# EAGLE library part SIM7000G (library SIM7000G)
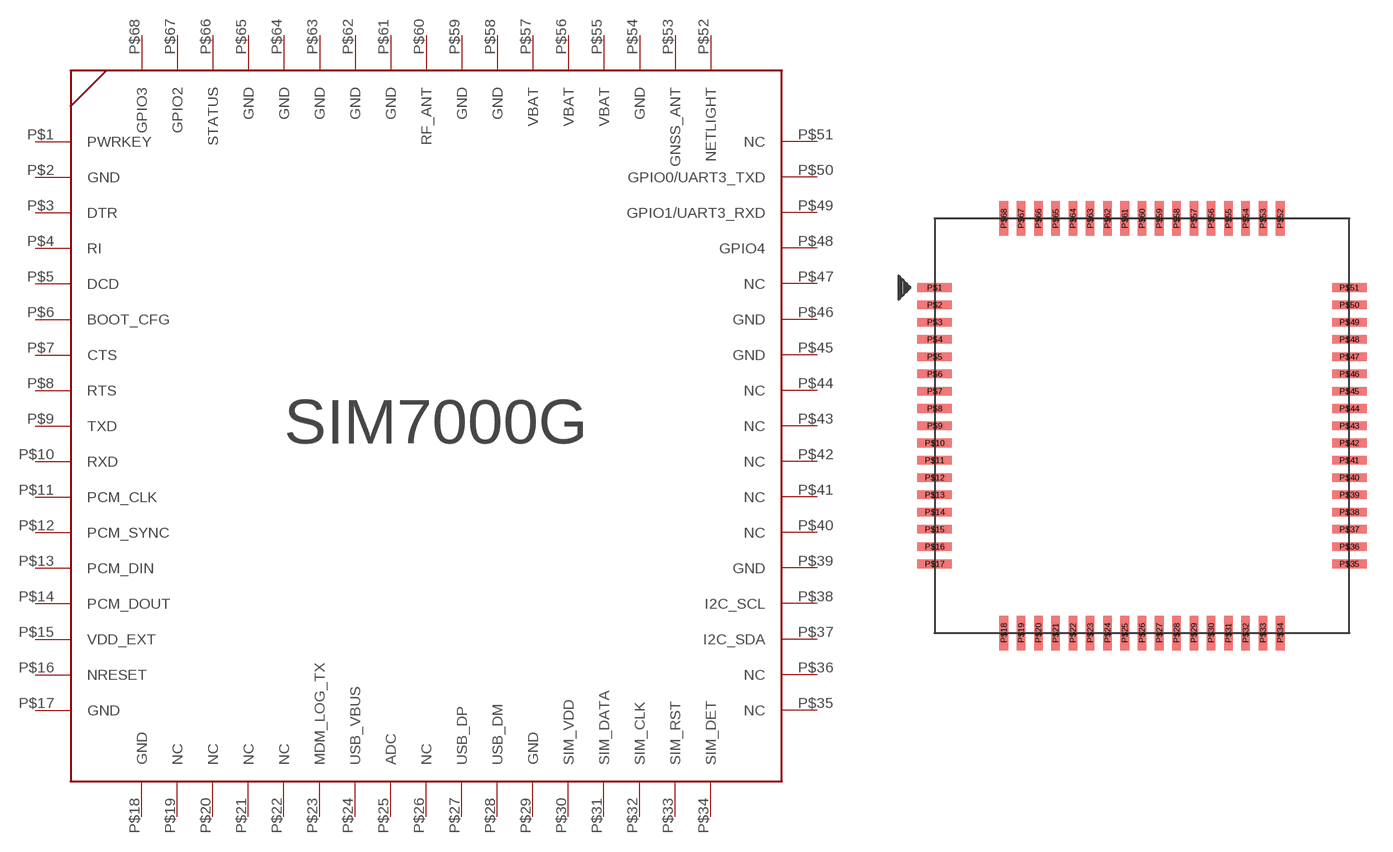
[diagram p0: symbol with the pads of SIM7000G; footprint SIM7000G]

Designator prefix -

## SIM7000G (CHECK_PRICES: https://www.snapeda.com/parts/SIM7000G/SIMCom/view-part/?ref=eda; DESCRIPTION: 802.15.4 Cat-M, Cat-NB, EDGE, GPRS, LPWA Transceiver Module 850MHz, 900MHz, 1.8GHz, 1.9GHz Antenna Not Included Surface Mount; MF: SIMCom Wireless Solutions Limited; MP: SIM7000G; PACKAGE: None; PURCHASE-URL: https://www.snapeda.com/api/url_track_click_mouser/?unipart_id=12130268&manufacturer=SIMCom Wireless Solutions Limited&part_name=SIM7000G&search_term=sim7000g; SNAPEDA_LINK: https://www.snapeda.com/parts/SIM7000G/SIMCom/view-part/?ref=snap)  [SIM7000G]
P$1  PWRKEY
P$2  GND
P$3  DTR
P$4  RI
P$5  DCD
P$6  BOOT_CFG
P$7  CTS
P$8  RTS
P$9  TXD
P$10  RXD
P$11  PCM_CLK
P$12  PCM_SYNC
P$13  PCM_DIN
P$14  PCM_DOUT
P$15  VDD_EXT
P$16  NRESET
P$17  GND
P$18  GND
P$19  NC
P$20  NC
P$21  NC
P$22  NC
P$23  MDM_LOG_TX
P$24  USB_VBUS
P$25  ADC
P$26  NC
P$27  USB_DP
P$28  USB_DM
P$29  GND
P$30  SIM_VDD
P$31  SIM_DATA
P$32  SIM_CLK
P$33  SIM_RST
P$34  SIM_DET
P$35  NC
P$36  NC
P$37  I2C_SDA
P$38  I2C_SCL
P$39  GND
P$40  NC
P$41  NC
P$42  NC
P$43  NC
P$44  NC
P$45  GND
P$46  GND
P$47  NC
P$48  GPIO4
P$49  GPIO1/UART3_RXD
P$50  GPIO0/UART3_TXD
P$51  NC
P$52  NETLIGHT
P$53  GNSS_ANT
P$54  GND
P$55  VBAT
P$56  VBAT
P$57  VBAT
P$58  GND
P$59  GND
P$60  RF_ANT
P$61  GND
P$62  GND
P$63  GND
P$64  GND
P$65  GND
P$66  STATUS
P$67  GPIO2
P$68  GPIO3

## Footprint SIM7000G (pad centres in mm)
smd 2 x 0.5: P$1 -12,8; P$2 -12,7; P$3 -12,6; P$4 -12,5; P$5 -12,4; P$6 -12,3; P$7 -12,2; P$8 -12,1; P$9 -12,0; P$10 -12,-1; P$11 -12,-2; P$12 -12,-3; P$13 -12,-4; P$14 -12,-5; P$15 -12,-6; P$16 -12,-7; P$17 -12,-8; P$35 12,-8; P$36 12,-7; P$37 12,-6; P$38 12,-5; P$39 12,-4; P$40 12,-3; P$41 12,-2; P$42 12,-1; P$43 12,0; P$44 12,1; P$45 12,2; P$46 12,3; P$47 12,4; P$48 12,5; P$49 12,6; P$50 12,7; P$51 12,8
smd 0.5 x 2: P$18 -8,-12; P$19 -7,-12; P$20 -6,-12; P$21 -5,-12; P$22 -4,-12; P$23 -3,-12; P$24 -2,-12; P$25 -1,-12; P$26 0,-12; P$27 1,-12; P$28 2,-12; P$29 3,-12; P$30 4,-12; P$31 5,-12; P$32 6,-12; P$33 7,-12; P$34 8,-12; P$52 8,12; P$53 7,12; P$54 6,12; P$55 5,12; P$56 4,12; P$57 3,12; P$58 2,12; P$59 1,12; P$60 0,12; P$61 -1,12; P$62 -2,12; P$63 -3,12; P$64 -4,12; P$65 -5,12; P$66 -6,12; P$67 -7,12; P$68 -8,12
